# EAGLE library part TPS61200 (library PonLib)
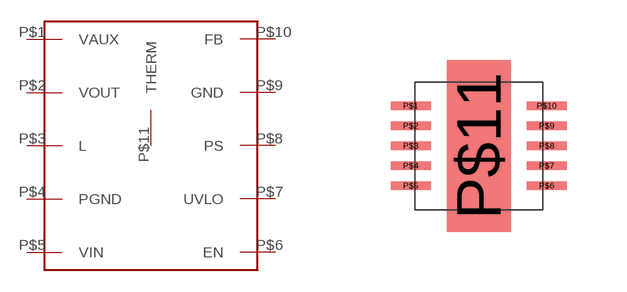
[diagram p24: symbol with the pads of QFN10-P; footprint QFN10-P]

Designator prefix -

## TPS61200  [QFN10-P]
P$1  VAUX
P$2  VOUT
P$3  L
P$4  PGND
P$5  VIN
P$6  EN
P$7  UVLO
P$8  PS
P$9  GND
P$10  FB
P$11  THERM

## Footprint QFN10-P (pad centres in mm)
smd 1 x 0.22: P$1 -1.7,1; P$2 -1.7,0.5; P$3 -1.7,0; P$4 -1.7,-0.5; P$5 -1.7,-1; P$6 1.7,-1; P$7 1.7,-0.5; P$8 1.7,0; P$9 1.7,0.5; P$10 1.7,1
smd 1.6 x 4.3: P$11 0,0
